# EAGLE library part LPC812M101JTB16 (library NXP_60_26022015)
32-bit ARM Cortex-M0+ microcontroller The LPC81xM are an ARM Cortex-M0+ based, low-cost 32-bit MCU family operating at CPU frequencies of up to 30 MHz. The LPC81xM support up to 16 kB of flash memory and 4 kB of SRAM. The peripheral complement of the LPC81xM includes a CRC engine, one I 2 C-bus interface, up to three USARTs, up to two SPI interfaces, one multi-rate timer, self wake-up timer, and state-configurable timer, one comparator, function-configurable I/O ports through a switch matrix, an input pattern match engine, and up to 18 general-purpose I/O pins. AAL Eindhoven MK
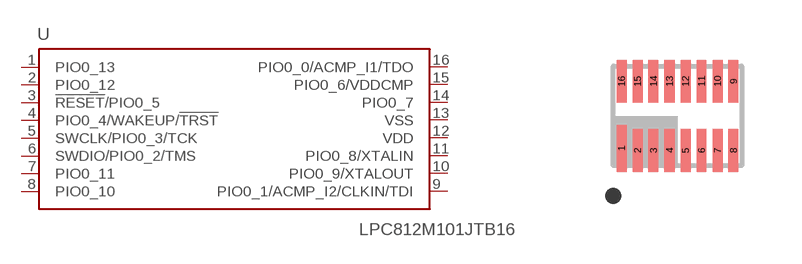
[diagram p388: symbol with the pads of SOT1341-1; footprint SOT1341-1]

Designator prefix U

## LPC812M101JTB16  [SOT1341-1]
1  PIO0_13
2  PIO0_12
3  !RESET!/PIO0_5
4  PIO0_4/WAKEUP/!TRST!
5  SWCLK/PIO0_3/TCK
6  SWDIO/PIO0_2/TMS
7  PIO0_11
8  PIO0_10
9  PIO0_1/ACMP_I2/CLKIN/TDI
10  PIO0_9/XTALOUT
11  PIO0_8/XTALIN
12  VDD  pwr
13  VSS  pwr
14  PIO0_7
15  PIO0_6/VDDCMP
16  PIO0_0/ACMP_I1/TDO

## Footprint SOT1341-1 (pad centres in mm)
SOT1341-1 XSON16: plastic extremely thin small outline package; no leads; 16 terminals; body 2.5 x 3.2 x 0.5 mm JEDEC: MO-252 IEC: -- JEITA: --date: 2014-01-21 REMARK: This is not an official NXP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
smd 0.25 x 1.17: 1 -1.4,-0.815
smd 0.25 x 1.07: 2 -1,-0.865; 3 -0.6,-0.865; 4 -0.2,-0.865; 5 0.2,-0.865; 6 0.6,-0.865; 7 1,-0.865; 8 1.4,-0.865; 9 1.4,0.865; 10 1,0.865; 11 0.6,0.865; 12 0.2,0.865; 13 -0.2,0.865; 14 -0.6,0.865; 15 -1,0.865; 16 -1.4,0.865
